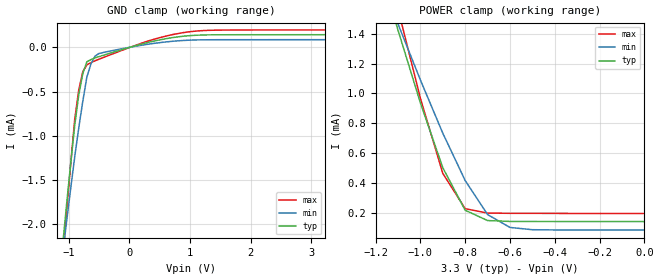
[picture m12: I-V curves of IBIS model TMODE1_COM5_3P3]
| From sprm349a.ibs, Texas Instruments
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|TMODE4_IND5_3P3BUFFER IN NORMAL MODE WITH INDTEMP AT 5PERCENT VDDS
|   Model Cell TMODE1_COM5_3P3
|TMODE1_COM5_3P3
[Model]   TMODE1_COM5_3P3
Model_type   Input
Polarity   Non-Inverting
Vinl =  0.8V
Vinh =  2V
C_comp   0.5121187p   0.4653713p   0.5743862p
[Model Spec]
Vinl   0.8V   0.8V   0.8V
Vinh   2V   2V   2V
[Temperature Range]   25   105   0
[Voltage Range]   3.3   3.14   3.47
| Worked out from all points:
|   GND clamp passes 1 mA (typ) near -0.92 V on its own axis
|   POWER clamp passes 1 mA (typ) near -1.01 V on its own axis
[POWER_clamp]
|   voltage   I(typ)   I(min)   I(max)
-3.3V     12.69mA    10.13mA    15.25mA
-1.1V     1.424mA    1.466mA    1.566mA
-1.067V   1.262mA    1.341mA    1.367mA
-1V       937.2uA    1.091mA    968.1uA
-900mV    503.7uA    734.6uA    465.6uA
-800mV    218.8uA    417.5uA    229.2uA
-700mV    149.8uA    190uA      199.9uA
-600mV    144uA      103.7uA    198.3uA
-500mV    143.6uA    88.62uA    198uA
-11.55fV  143uA      86.7uA     197uA
[GND_clamp]
|   voltage   I(typ)   I(min)   I(max)
-3.3V     -19.06mA   -15.34mA   -22.43mA
-1.1V     -2.241mA   -2.339mA   -2.416mA
-1.033V   -1.769mA   -1.963mA   -1.852mA
-900mV    -882.6uA   -1.238mA   -813.9uA
-833.3mV  -536.3uA   -908.9uA   -480.5uA
-766.7mV  -296.3uA   -608.4uA   -275.2uA
-700mV    -162.6uA   -336.1uA   -197.8uA
-566.7mV  -119.5uA   -100.2uA   -152uA
-500mV    -104.7uA   -69.34uA   -133.8uA
300mV     54.16uA    34.42uA    69.63uA
966.7mV   130.5uA    80.39uA    173.7uA
3.233V    143uA      86.74uA    196.8uA
